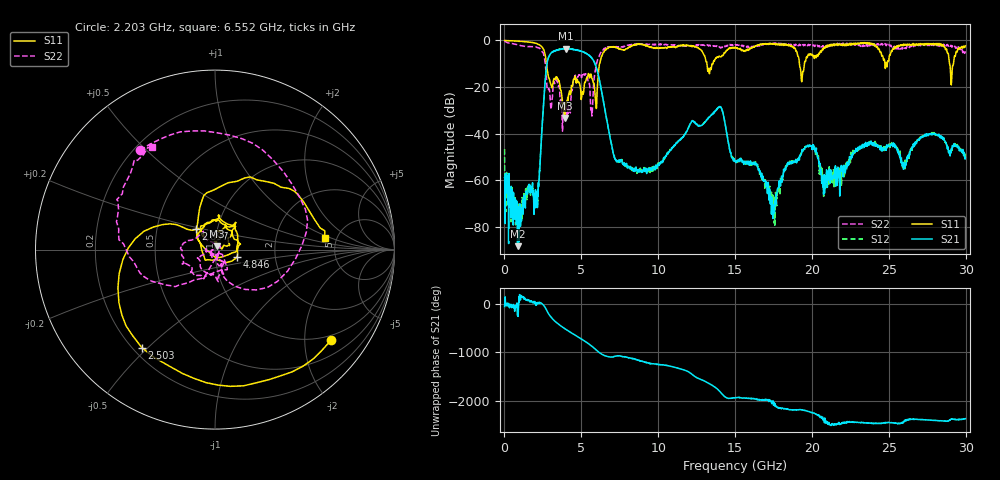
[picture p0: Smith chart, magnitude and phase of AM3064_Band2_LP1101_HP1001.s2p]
# Hz S DB R 50.0
!freq dBS11 angS11 dBS21 angS21 dBS12 angS12 dBS22 angS22
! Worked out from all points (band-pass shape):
!   1600 points, 10 MHz to 29.98 GHz, reference 50 ohm
!   highest |S21| = -3.47 dB at 4.002 GHz (marker M1); lowest = -88.2 dB at 853.5 MHz (marker M2)
!   |S21| within 3 dB of the highest: 2.927 GHz to 5.499 GHz (2.572 GHz wide, 61 % of centre); 5.505587 GHz to 5.527158 GHz (21.57 MHz wide, 0.391 % of centre)
!   lowest |S11| = -33.3 dB at 3.909 GHz (marker M3), VSWR 1.04, Z = 51 + j1.96 ohm
!   |S11| at or under -10 dB: 2.732 GHz to 6.19 GHz (3.458 GHz wide, 77.5 % of centre); 13.17 GHz to 13.5 GHz (333.7 MHz wide, 2.5 % of centre); 19.18 GHz to 19.51 GHz (325.7 MHz wide, 1.68 % of centre)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
!   |S22| runs from -38.9 to -0.2 dB; largest |S21 - S12| = 0.02
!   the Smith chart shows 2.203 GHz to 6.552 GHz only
!   S11 on the Smith chart (normalised r, x): 2.203 GHz: 0.86, -2.66; 2.503 GHz: 0.24, -0.48; 2.897 GHz: 0.79, +0.19; 4.846 GHz: 1.27, -0.11; 6.552 GHz: 4.01, +0.83
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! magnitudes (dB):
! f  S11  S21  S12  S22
! 10 MHz  0.0  -58.8  -46.6  -0.2
! 853.5 MHz  -0.3  -88.2  -78.3  -1.9
! 2.203 GHz  -1.7  -60.9  -62.3  -3.2
! 2.503 GHz  -3.3  -31.3  -31.3  -5.2
! 2.897 GHz  -16.2  -6.8  -6.8  -20.6
! 3.909 GHz  -33.3  -3.7  -3.5  -31.8
! 4.002 GHz  -26.6  -3.5  -3.6  -29.1
! 4.846 GHz  -17.9  -4.3  -4.3  -14.7
! 5.015 GHz  -24.4  -4.7  -4.7  -15.9
! 5.671 GHz  -16.0  -7.5  -7.4  -30.6
! 5.952 GHz  -27.3  -11.0  -11.1  -11.0
! 6.552 GHz  -4.2  -30.2  -30.3  -3.4
! 7.283 GHz  -3.2  -51.5  -52.0  -2.7
! 10 GHz  -3.3  -53.0  -53.1  -1.8
! 13.97 GHz  -6.7  -28.7  -28.5  -2.8
! 15 GHz  -3.0  -51.8  -51.7  -1.9
! 17.5 GHz  -1.5  -73.1  -71.2  -1.2
! 19.99 GHz  -6.0  -45.6  -45.4  -1.8
! 20.89 GHz  -2.5  -58.8  -61.3  -2.8
! 25 GHz  -8.5  -44.8  -44.4  -1.7
! 29.08 GHz  -17.8  -46.5  -46.1  -2.5
! 29.98 GHz  -2.3  -50.2  -48.7  -4.7
